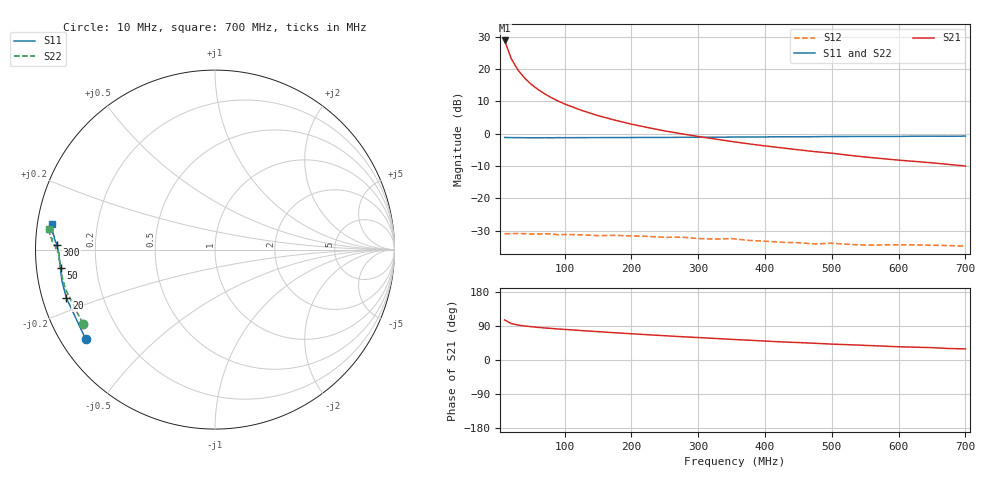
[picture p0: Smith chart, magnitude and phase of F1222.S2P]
! Date: Tue Aug 08 10:23:29 1995
# MHZ  S  MA  R  50.0000
!  POLYFET RF DEVICES
!  F1222
!  S PARAMETERS
!  VDS=12.5V, IDQ=400mA
!FREQ  S11MAG S11ANG S21MAG S21ANG S12MAG S12ANG S22MAG S22ANG
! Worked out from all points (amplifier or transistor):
!   34 points, 10 MHz to 700 MHz, reference 50 ohm
!   highest |S21| = 28.9 dB at 10 MHz (marker M1)
!   |S21| within 3 dB of that: start of sweep to 15.29 MHz
!   unconditionally stable (mu >= 1): 433.9 MHz to end of sweep
!   at 60 MHz: K = 0.13, MSG = 22.4 dB, |S12| = -31.0 dB
!   at 300 MHz: K = 0.67, MSG = 15.8 dB, |S12| = -32.4 dB
!   at 700 MHz: K = 1.44, MAG = 8.5 dB, |S12| = -34.8 dB
!   S11 on the Smith chart (normalised r, x): 10 MHz: 0.07, -0.31; 20 MHz: 0.07, -0.16; 50 MHz: 0.07, -0.06; 300 MHz: 0.06, +0.02; 700 MHz: 0.04, +0.08
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10  0.8764 -145.3  27.8 105.7  0.02832 15.4  0.8441 -150.8
20  0.871 -162.0  14.48 96.1  0.02851 7.7  0.8618 -165.3
30  0.8704 -168.1  9.691 92.4  0.02859 4.5  0.8655 -170.1
40  0.8687 -171.2  7.277 89.8  0.02841 3.2  0.8666 -172.7
50  0.8664 -173.2  5.81 87.8  0.02807 2.5  0.8684 -174.3
60  0.8673 -174.5  4.841 86.1  0.02808 1.1  0.8653 -175.3
70  0.8686 -175.4  4.149 84.6  0.02835 0.2  0.8688 -175.9
80  0.8668 -176.2  3.621 83.3  0.02805 0.2  0.8699 -176.6
90  0.8705 -176.8  3.211 81.9  0.02732 0.2  0.8664 -177.0
100  0.8689 -177.1  2.888 80.7  0.0276 -0.7  0.8685 -177.3
125  0.8705 -178.2  2.304 77.7  0.02729 -0.7  0.8703 -177.9
150  0.8714 -178.9  1.908 74.8  0.02649 -3.0  0.8701 -178.8
175  0.8738 -179.4  1.625 71.9  0.02676 -3.2  0.8776 -179.2
200  0.8746 -179.9  1.408 69.3  0.02621 -3.0  0.8768 -179.4
250  0.8778 179.1  1.105 64.0  0.02493 -2.5  0.885 179.7
300  0.8825 178.2  0.9065 59.3  0.02392 -2.4  0.8904 179.0
350  0.8884 177.3  0.7598 54.5  0.02389 -2.3  0.8926 178.4
375  0.8912 176.9  0.6995 52.3  0.02237 -0.3  0.899 177.8
475  0.9006 175.2  0.5281 44.1  0.0197 7.0  0.9091 176.8
500  0.9063 174.3  0.4999 41.9  0.02027 7.7  0.9101 176.2
600  0.9093 172.9  0.3905 34.9  0.01908 16.5  0.9216 174.9
700  0.9208 171.0  0.3166 29.4  0.0182 28.0  0.9342 172.9
